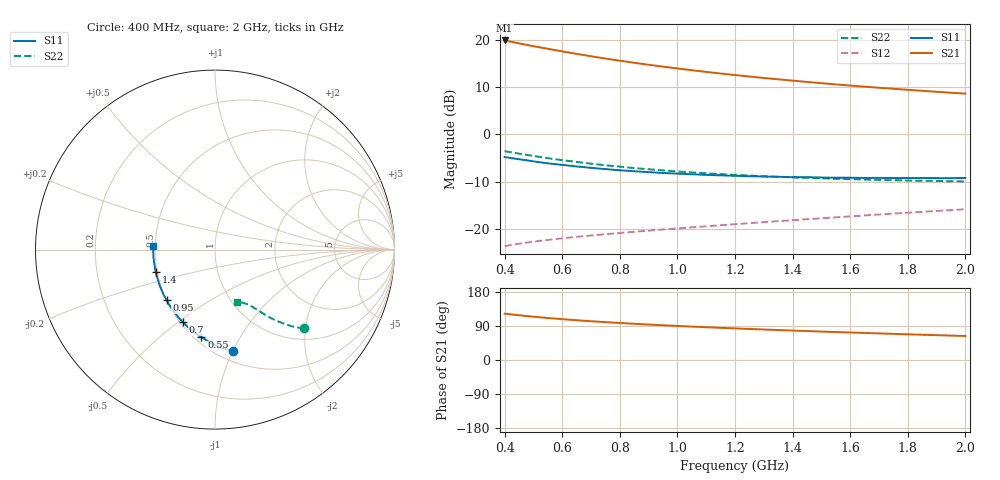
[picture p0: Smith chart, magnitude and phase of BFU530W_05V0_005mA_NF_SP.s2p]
! Filename:  P:\Prog\Test\Noise\ATS_data\Testdata_Net\06 Compressed Noise after Statistics\BFU530W_APM2013_09_A05_05p0V_005mA_NF_CM01_D.sf
! Date/Time: Tue 26/Mar/2013 18:06:05
! BFU530W_APM2013_09_A05_05p0V_1to25mA_NF_CM01_Bias4_R.sf
! Noise Parameter Data File
! BFU530W_APM2013_09_A05_05p0V_1to25mA_NF_CM01
! Date/time: Thu Mar 21 20:31:54 2013
! VAR V_out= 5.000000
! VAR I_out= 4.990000
! VAR V_in= 0.817700
! VAR I_in= 0.052005
! Device data file deembeded for feedlines and parallel
! Original file: \06 Compressed Noise after Statistics\BFU530W_APM2013_09_A05_05p0V_005mA_NF_CM01_R.sf
! Feed-files: PR019V01_070313_Feed1.s2p, PR019V01_070313_Feed2.s2p
! Parallel-file: PR019V01_070313_Par.s2p
# MHz S MA R 50
!  Freq-MHz  S11-mag  S11-arg  S21-mag  S21-arg  S12-mag  S12-arg  S22-mag  S22-arg
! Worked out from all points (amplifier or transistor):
!   37 points, 400 MHz to 2 GHz, reference 50 ohm
!   highest |S21| = 19.9 dB at 400 MHz (marker M1)
!   |S21| within 3 dB of that: start of sweep to 665.5 MHz
!   unconditionally stable (mu >= 1): 1.734 GHz to end of sweep
!   at 500 MHz: K = 0.51, MSG = 20.7 dB, |S12| = -22.7 dB
!   at 1.1 GHz: K = 0.86, MSG = 16.3 dB, |S12| = -19.5 dB
!   at 2 GHz: K = 1.02, MAG = 11.4 dB, |S12| = -15.9 dB
!   lowest NFmin = 0.58 dB at 440 MHz
!   S11 on the Smith chart (normalised r, x): 400 MHz: 0.59, -1.00; 550 MHz: 0.54, -0.70; 700 MHz: 0.52, -0.52; 950 MHz: 0.50, -0.33; 1.4 GHz: 0.49, -0.14; 2 GHz: 0.49, +0.02
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400  0.5754 -80.0  9.857 122.3  0.06549 56.1  0.6633 -41.4
420  0.5622 -82.8  9.583 120.5  0.06718 55.5  0.6476 -42.4
440  0.5506 -85.5  9.319 118.8  0.06874 54.9  0.6322 -43.4
480  0.5288 -90.6  8.809 115.8  0.07165 54.0  0.6042 -45.0
500  0.5176 -93.2  8.575 114.3  0.07301 53.6  0.5904 -45.7
550  0.4934 -98.9  8.044 110.8  0.0762 53.0  0.5597 -47.3
600  0.4747 -104.4  7.557 107.7  0.07933 52.5  0.5326 -48.6
650  0.4573 -109.3  7.104 105.0  0.08221 52.1  0.5102 -49.8
700  0.4415 -114.1  6.707 102.3  0.08497 52.0  0.4892 -50.9
750  0.4288 -118.4  6.341 100.0  0.08767 52.0  0.4704 -51.7
800  0.4163 -122.6  6.016 97.7  0.09041 52.1  0.455 -52.6
850  0.4067 -126.7  5.72 95.5  0.09305 52.2  0.4396 -53.3
950  0.39 -133.8  5.207 91.7  0.09836 52.6  0.4154 -54.7
1050  0.3779 -140.4  4.772 88.2  0.1036 53.2  0.3952 -55.9
1150  0.3678 -146.6  4.404 84.9  0.1091 53.7  0.3789 -57.0
1200  0.3637 -149.2  4.245 83.4  0.1119 54.1  0.3728 -57.6
1300  0.3574 -154.6  3.953 80.5  0.1175 54.7  0.3601 -58.6
1400  0.3523 -159.6  3.701 77.7  0.1233 55.2  0.3501 -59.8
1500  0.3492 -164.0  3.479 75.0  0.1293 55.7  0.3425 -61.1
1650  0.3454 -170.5  3.195 71.4  0.1384 56.4  0.3321 -62.8
1750  0.3448 -174.3  3.037 69.0  0.1449 56.8  0.3272 -64.1
2000  0.3456 176.7  2.697 63.4  0.1611 57.4  0.3177 -67.7
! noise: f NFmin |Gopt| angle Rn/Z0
400  0.6262  0.1593  32.79  0.1042
460  0.6146  0.1575  40.8  0.1013
600  0.6387  0.176  45.14  0.109
800  0.6693  0.1704  68.95  0.0982
1000  0.6891  0.1865  81.6  0.0967
1200  0.7502  0.202  95.71  0.0915
1400  0.7609  0.2243  112.9  0.0822
1600  0.7581  0.234  127.7  0.0761
1800  0.8255  0.2454  144.7  0.0679
2000  0.8794  0.2605  155.7  0.065
